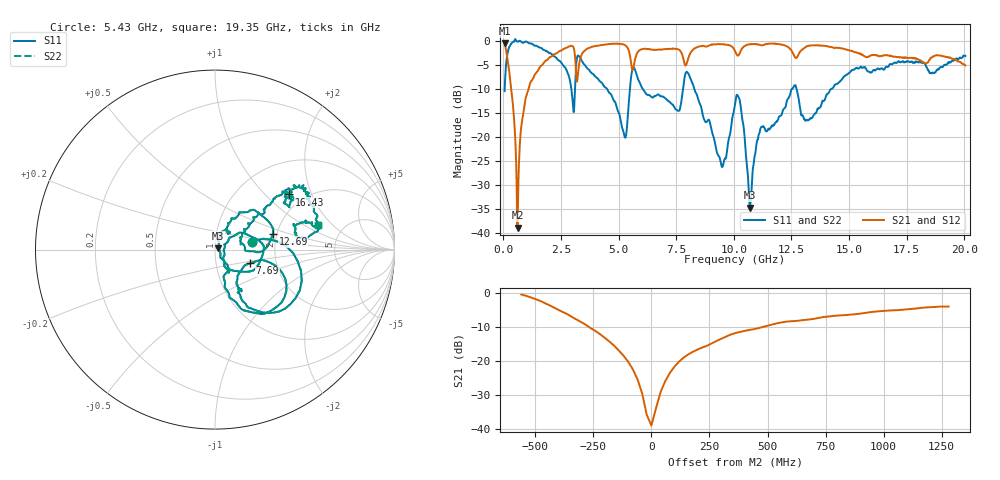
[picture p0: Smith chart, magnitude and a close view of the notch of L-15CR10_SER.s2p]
#	mhz	s	ma	r	50
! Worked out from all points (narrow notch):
!   1001 points, 50 MHz to 20.05 GHz, reference 50 ohm
!   highest |S21| = -0.58 dB at 50 MHz (marker M1); lowest = -38.9 dB at 610 MHz (marker M2)
!   notch at M2: 37.0 dB deep, 215 MHz wide at half that depth
!   lowest |S11| = -34.8 dB at 10.69 GHz (marker M3), VSWR 1.04, Z = 51.6 + j0.854 ohm
!   |S11| at or under -10 dB: 6.037 GHz to 7.794 GHz (1.757 GHz wide, 25.4 % of centre); 8.279 GHz to 12.54 GHz (4.264 GHz wide, 41 % of centre); 12.72 GHz to 14.27 GHz (1.55 GHz wide, 11.5 % of centre)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
!   |S22| runs from -34.8 to 0.3 dB; largest |S21 - S12| = 0
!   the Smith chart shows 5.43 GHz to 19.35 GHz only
!   S11 on the Smith chart (normalised r, x): 5.43 GHz: 1.51, +0.14; 7.69 GHz: 1.46, -0.23; 12.69 GHz: 1.90, +0.38; 16.43 GHz: 1.67, +1.40; 19.35 GHz: 3.22, +1.37
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50  0.2972 70.4  0.9358 -16.7  0.9358 -16.7  0.2972 70.4
610  0.9743 -2.6  0.0113 5.3  0.0113 5.3  0.9743 -2.6
1270  0.9178 -28.3  0.3975 63.6  0.3975 63.6  0.9178 -28.3
3010  0.223 -56.7  0.8688 4.5  0.8688 4.5  0.223 -56.7
3390  0.6184 -51.7  0.7083 30.6  0.7083 30.6  0.6184 -51.7
5230  0.1055 -49.0  0.9031 -8.4  0.9031 -8.4  0.1055 -49.0
5430  0.2105 12.1  0.8008 -18.6  0.8008 -18.6  0.2105 12.1
5650  0.5239 -31.1  0.5303 5.9  0.5303 5.9  0.5239 -31.1
6730  0.2748 -57.3  0.8041 -4.0  0.8041 -4.0  0.2748 -57.3
7690  0.2096 -21.3  0.7705 -17.4  0.7705 -17.4  0.2096 -21.3
8030  0.4518 -52.0  0.6638 4.6  0.6638 4.6  0.4518 -52.0
9510  0.04873 -1.8  0.9143 -16.1  0.9143 -16.1  0.04873 -1.8
10050  0.2166 19.1  0.7791 -25.1  0.7791 -25.1  0.2166 19.1
10310  0.1957 -39.0  0.7901 -10.2  0.7901 -10.2  0.1957 -39.0
10690  0.01821 27.0  0.9142 -16.9  0.9142 -16.9  0.01821 27.0
11170  0.1239 62.1  0.8935 -22.6  0.8935 -22.6  0.1239 62.1
12690  0.3342 15.3  0.6574 -32.3  0.6574 -32.3  0.3342 15.3
13390  0.1558 25.1  0.8906 -31.6  0.8906 -31.6  0.1558 25.1
16430  0.5138 36.8  0.6924 -47.2  0.6924 -47.2  0.5138 36.8
16730  0.5445 38.0  0.6963 -48.8  0.6963 -48.8  0.5445 38.0
19350  0.588 13.7  0.6628 -65.4  0.6628 -65.4  0.588 13.7
20050  0.6903 2.3  0.5512 -78.1  0.5512 -78.1  0.6903 2.3
